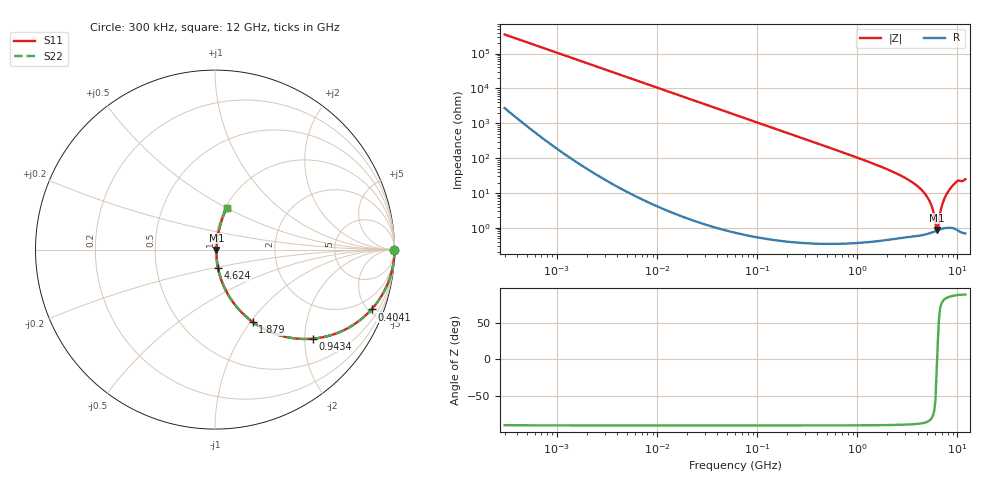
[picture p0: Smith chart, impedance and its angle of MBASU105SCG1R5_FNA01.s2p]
! MBASU105SCG1R5_FNA01  S-PARAMETER MODEL  ( Standard Model )
! Model Generated by TAIYO YUDEN Corporation (http://www.ty-top.com)
! Version 1.0
! TAIYO YUDEN Control No. 230609
! Copyright(c) 2023 TAIYO YUDEN CO.,LTD. All Rights Reserved.
! Product Description (link to TY-COMPAS)
! https://ds.yuden.co.jp/TYCOMPAS/or/detail?pn=MBASU105SCG1R5BFNA01&u=M
! Products Name : Multilayer Ceramic Capacitors
! Characteristics :
!  Capacitance : 1.5 [pF] , Rated Voltage : 50 [V] , TCC : CG / C0G
!  Case Size : 1.0 x 0.5 / 0.039 x 0.02 [mm/inch] , Thickness : 0.5 / 0.02 [mm/inch]
!  (Conditions: Temperature = 25 [degC] , DC Bias Voltage = 0 [V])
! External Node Assignments :
!  1  o---| |---o  2
! GND o---------o GND
! Frequency Range : 0.3MHz  -  12000MHz  [ 401 STEP ]
# MHZ S RI R 50
! Freq[MHz].  S11 Real  S11 Imag  S21 Real  S21 Imag  S12 Real  S12 Imag  S22 Real  S22 Imag
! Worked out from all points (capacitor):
!   401 points, 300 kHz to 12 GHz, reference 50 ohm
!   read as one part in series: C = 1.5 pF near 316.3 kHz
!   lowest |Z| = 865 mohm at 6.188 GHz (marker M1)
!   series resonance near 6.259 GHz, so ESL is about 430 pH
!   S11 on the Smith chart (normalised r, x): 300 kHz: open; 404.1 MHz: 1.01, -5.23; 943.4 MHz: 1.01, -2.20; 1.879 GHz: 1.01, -1.03; 4.624 GHz: 1.01, -0.21; 12 GHz: 1.01, +0.50
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0.3  1 -0.000283  2.27e-06 0.000283  2.27e-06 0.000283  1 -0.000283
1.769972  1 -0.00167  4.49e-06 0.00167  4.49e-06 0.00167  1 -0.00167
10.44266  0.9999 -0.00984  0.000101 0.00984  0.000101 0.00984  0.9999 -0.00984
60  0.9968 -0.0564  0.00321 0.0564  0.00321 0.0564  0.9968 -0.0564
155.7172  0.9788 -0.1437  0.0212 0.1437  0.0212 0.1437  0.9788 -0.1437
353.9943  0.899 -0.3008  0.101 0.3008  0.101 0.3008  0.899 -0.3008
404.1309  0.872 -0.3334  0.128 0.3334  0.128 0.3334  0.872 -0.3334
943.3804  0.5469 -0.4961  0.4531 0.4961  0.4531 0.4961  0.5469 -0.4961
1878.541  0.2108 -0.4036  0.7892 0.4036  0.7892 0.4036  0.2108 -0.4036
2088.533  0.1716 -0.372  0.8284 0.372  0.8284 0.372  0.1716 -0.372
3364.605  0.0524 -0.2108  0.9476 0.2108  0.9476 0.2108  0.0524 -0.2108
4623.766  0.0167 -0.1011  0.9833 0.1011  0.9833 0.1011  0.0167 -0.1011
5420.343  0.00939 -0.0472  0.9906 0.0472  0.9906 0.0472  0.00939 -0.0472
6026.253  0.0081 -0.0116  0.9919 0.0116  0.9919 0.0116  0.0081 -0.0116
6188.031  0.00821 -0.00248  0.9918 0.00248  0.9918 0.00248  0.00821 -0.00248
6354.153  0.00845 0.0033  0.9915 -0.0033  0.9915 -0.0033  0.00845 0.0033
6524.734  0.00882 0.0115  0.9912 -0.0115  0.9912 -0.0115  0.00882 0.0115
7064.448  0.0115 0.0458  0.9885 -0.0458  0.9885 -0.0458  0.0115 0.0458
7254.098  0.0129 0.0573  0.9871 -0.0573  0.9871 -0.0573  0.0129 0.0573
8064.993  0.0214 0.1058  0.9786 -0.1058  0.9786 -0.1058  0.0214 0.1058
9708.23  0.0483 0.1935  0.9517 -0.1935  0.9517 -0.1935  0.0483 0.1935
12000  0.0641 0.2314  0.9359 -0.2314  0.9359 -0.2314  0.0641 0.2314
